FUNCTION_BLOCK Example06_sync //4x3 flyways, 4 xbots - get xbot prop, set xbot prop, sync move
VAR_INPUT
	Execute : BOOL;
END_VAR
VAR_OUTPUT
	Done : BOOL;
END_VAR
VAR_IN_OUT
	PM_Controller : PMControllerType;	// the planar motor controller to use
END_VAR
VAR
	xbotID_array78 : ARRAY[0..77] OF USINT;
	PosX_array78 : ARRAY[0..77] OF REAL;
	PosY_array78 : ARRAY[0..77] OF REAL;
	PMC_AutoDrivingMotion1 : PMC_AutoDrivingMotion;
	xbotID_array14 : ARRAY[0..13] OF USINT;
	xbotprop_array14 : ARRAY[0..13] OF USINT;
	propvalue_array14 : ARRAY[0..13] OF REAL;
	xbotID_array4 : ARRAY[0..3] OF USINT;
	endvel_4 : ARRAY[0..3] OF REAL;
	posx_4 : ARRAY[0..3] OF REAL;
	posy_4 : ARRAY[0..3] OF REAL;
	maxacc_4 : ARRAY[0..3] OF REAL;
	maxvel_4 : ARRAY[0..3] OF REAL;
	PMC_SyncMotion1 : PMC_SyncMotion;
	PMC_SyncMotion2 : PMC_SyncMotion;
END_VAR

//4x3 flyways, 4 xbots - get xbot prop, set xbot prop, sync move

//async move to 60,60 300,60 540,60 780,60
xbotID_array78[0] := 1;xbotID_array78[1] := 2;xbotID_array78[2] := 3;xbotID_array78[3] := 4;
PosX_array78[0] := 0.060;PosX_array78[1] := 0.300;PosX_array78[2] := 0.540;PosX_array78[3] := 0.780;
PosY_array78[0] := 0.060;PosY_array78[1] := 0.060;PosY_array78[2] := 0.060;PosY_array78[3] := 0.060;
PMC_AutoDrivingMotion1(Execute := Execute,nXbots := 4,RoutingType := 0,ZoneID := 0,XbotID := xbotID_array78,PosX := PosX_array78,PosY := PosY_array78,PM_Controller := PM_Controller);

//sync move all xbots to top of flyways
xbotID_array4[0] := 1;xbotID_array4[1] := 2;xbotID_array4[2] := 3;xbotID_array4[3] := 4;
endvel_4[0] := 0.0;endvel_4[1] := 0.0;endvel_4[2] := 0.0;endvel_4[3] := 0.0;
posx_4[0] := 0.06;posx_4[1] := 0.30;posx_4[2] := 0.54;posx_4[3] := 0.78;
posy_4[0] := 0.66;posy_4[1] := 0.66;posy_4[2] := 0.66;posy_4[3] := 0.66;
maxacc_4[0] := 10;maxacc_4[1] := 10;maxacc_4[2] := 20;maxacc_4[3] := 20;
maxvel_4[0] := 1;maxvel_4[1] := 1;maxvel_4[2] := 2;maxvel_4[3] := 2;
PMC_SyncMotion1(Execute := PMC_AutoDrivingMotion1.Done,nXbots := 4,XbotID := xbotID_array4,PosX := posx_4,PosY := posy_4,EndVel := endvel_4,MaxVel := maxvel_4,MaxAcc := maxacc_4,PM_Controller := PM_Controller);

//sync move all xbots to bottom of flyways
xbotID_array4[0] := 1;xbotID_array4[1] := 2;xbotID_array4[2] := 3;xbotID_array4[3] := 4;
endvel_4[0] := 0.0;endvel_4[1] := 0.0;endvel_4[2] := 0.0;endvel_4[3] := 0.0;
posx_4[0] := 0.06;posx_4[1] := 0.30;posx_4[2] := 0.54;posx_4[3] := 0.78;
posy_4[0] := 0.06;posy_4[1] := 0.06;posy_4[2] := 0.06;posy_4[3] := 0.06;
maxacc_4[0] := 20;maxacc_4[1] := 20;maxacc_4[2] := 10;maxacc_4[3] := 10;
maxvel_4[0] := 2;maxvel_4[1] := 2;maxvel_4[2] := 1;maxvel_4[3] := 1;
PMC_SyncMotion2(Execute := PMC_SyncMotion1.Done,nXbots := 4,XbotID := xbotID_array4,PosX := posx_4,PosY := posy_4,EndVel := endvel_4,MaxVel := maxvel_4,MaxAcc := maxacc_4,PM_Controller := PM_Controller);

Done := PMC_SyncMotion2.Done;

END_FUNCTION_BLOCK
